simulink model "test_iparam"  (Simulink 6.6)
settings: Solver=ode45  StartTime=0.0  StopTime=10.0  RelTol=1e-3
libraries: sltpda x3

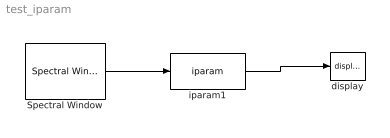
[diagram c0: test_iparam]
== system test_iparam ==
  Spectral Window : sltpda/AO class/Spectral Window  SystemSampleTime=-1  wname=Hanning  wlen=10  psll=0
  display : sltpda/AO class/display  Tag=display  SystemSampleTime=-1
  iparam1 : sltpda/AO class/iparam  SystemSampleTime=-1  key=Win
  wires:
  Spectral Window/1 -> iparam1/1
  iparam1/1 -> display/1
